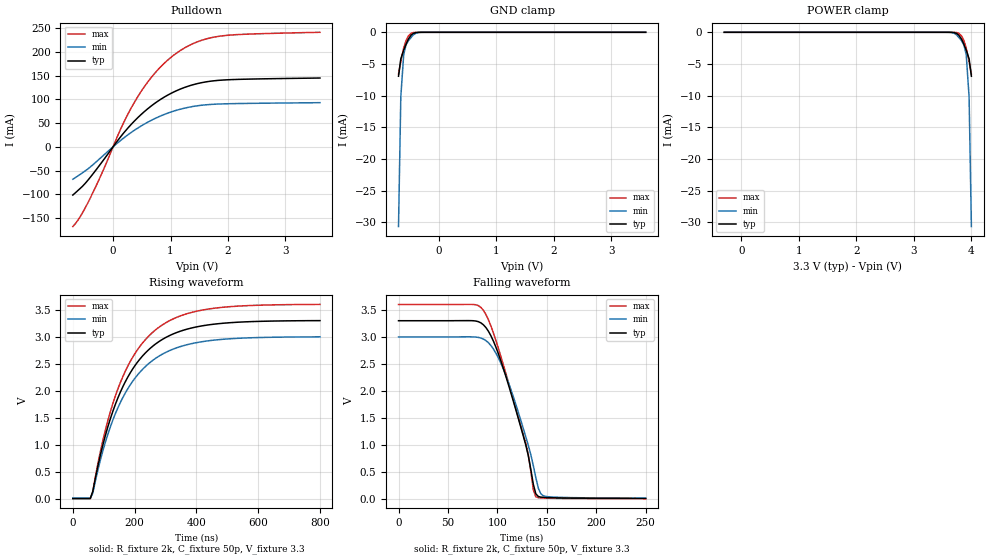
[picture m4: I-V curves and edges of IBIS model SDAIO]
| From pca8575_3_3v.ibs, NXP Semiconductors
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[Model]   SDAIO
Model_type I/O_open_drain
Enable Active-Low
Vinh=2.31
Vinl=0.99
Vref=3.3
Vmeas=1.65
Rref=2k
Cref=50p
C_comp   8p   7.8p   8.2p
[Temperature Range] 27   85   -40
[Voltage Range]   3.3   3   3.6
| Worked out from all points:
|   slope of the pulldown table from 0 to 0.495 V, typ, clamps not added: 7.2 ohm
|   GND clamp passes 1 mA (typ) near -0.52 V on its own axis
|   falling waveform, R_fixture 2k, C_fixture 50p, V_fixture 3.3: 20-80 % time 30.7ns typ, 30.3ns min, 32.7ns max; typ from 3.3 V to 0.011 V
|   rising waveform, R_fixture 2k, C_fixture 50p, V_fixture 3.3: 20-80 % time 142ns typ, 142ns min, 141ns max; typ from 0.01 V to 3.3 V
[Pulldown]
-700mV    -101.5mA   -68.23mA   -167.9mA
-570mV    -87.44mA   -57.86mA   -146.8mA
-400mV    -64.71mA   -42.87mA   -108.7mA
-180mV    -29.94mA   -19.38mA   -51.74mA
130mV     20.95mA    13.31mA    36.78mA
390mV     56.62mA    36.38mA    97.56mA
690mV     88.38mA    57.32mA    149.8mA
1.04V     114.5mA    74.62mA    191.5mA
1.43V     132mA      85.78mA    219.3mA
1.82V     139.8mA    90.04mA    232.4mA
2.3V      142.4mA    91.39mA    237.1mA
3.6V      144.9mA    92.99mA    241.2mA
[GND Clamp]
-700mV    -6.935mA   -30.66mA   -6.593mA
-660mV    -4.196mA   -10.18mA   -4.586mA
-610mV    -2.801mA   -3.515mA   -2.483mA
-570mV    -1.922mA   -2.007mA   -1.319mA
-530mV    -1.094mA   -1.347mA   -591uA
-480mV    -441.4uA   -796.7uA   -154.1uA
-440mV    -172.9uA   -393.1uA   -38.38uA
-350mV    -9.861uA   -39.84uA   -825nA
-270mV    -445.9nA   -2.659uA   -19.23nA
3.6V      201.4pA    372.1pA    187.3pA
[POWER Clamp]
-300mV    201.4pA    372.1pA    187.3pA
3.57V     -445.9nA   -2.659uA   -19.23nA
3.65V     -9.861uA   -39.84uA   -825nA
3.74V     -172.9uA   -393.1uA   -38.38uA
3.78V     -441.4uA   -796.7uA   -154.1uA
3.83V     -1.094mA   -1.347mA   -591uA
3.87V     -1.922mA   -2.007mA   -1.319mA
3.91V     -2.801mA   -3.515mA   -2.483mA
3.96V     -4.196mA   -10.18mA   -4.586mA
4V        -6.935mA   -30.66mA   -6.593mA
[Falling Waveform]
R_fixture=2k
C_fixture=50p
V_fixture=3.3
V_fixture_min=3
V_fixture_max=3.6
0s        3.3V       3V         3.6V
85.86ns   3.225V     2.961V     3.492V
95.96ns   2.924V     2.777V     3.075V
108.6ns   2.271V     2.286V     2.323V
128.8ns   996.3mV    1.148V     1.021V
136.4ns   271.5mV    615.6mV    170.8mV
138.9ns   95.93mV    396.3mV    40.68mV
143.9ns   35.42mV    97.24mV    21.23mV
149ns     28.14mV    47.53mV    16.82mV
250ns     11.05mV    16.24mV    6.693mV
[Rising Waveform]
R_fixture=2k
C_fixture=50p
V_fixture=3.3
V_fixture_min=3
V_fixture_max=3.6
0s        9.794mV    14.09mV    6.025mV
56.57ns   9.311mV    14.12mV    6.025mV
64.65ns   138.7mV    105.2mV    136.4mV
105.1ns   1.167V     1.044V     1.266V
153.5ns   1.971V     1.78V      2.148V
210.1ns   2.536V     2.297V     2.766V
274.7ns   2.894V     2.626V     3.157V
347.5ns   3.101V     2.816V     3.383V
444.4ns   3.223V     2.929V     3.516V
800ns     3.298V     2.998V     3.597V
[Ramp]
R_load=2k
dV/dt_r   1.974E+0/3.526E-9   1.971E+0/3.922E-9   1.977E+0/3.170E-9
dV/dt_f   1.973E+0/2.936E-8   1.969E+0/3.103E-8   1.976E+0/2.900E-8
|[End   SDAIO
